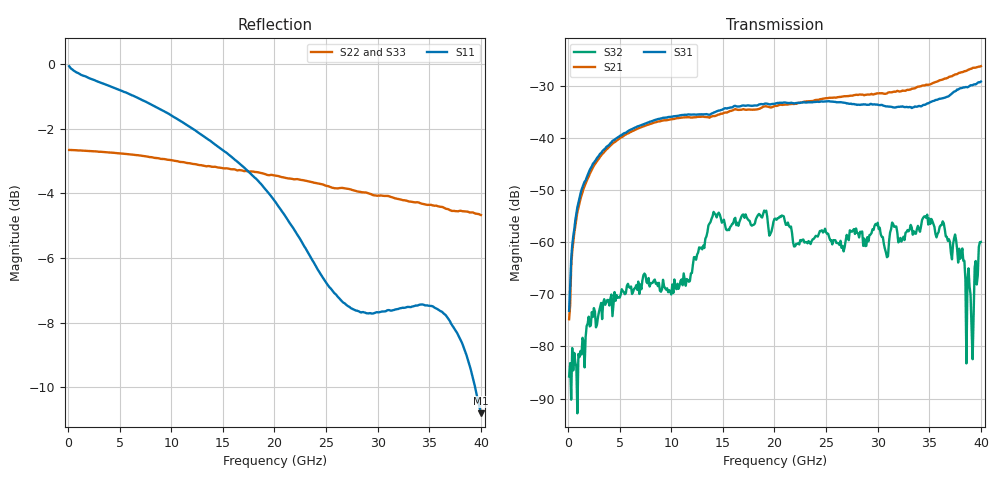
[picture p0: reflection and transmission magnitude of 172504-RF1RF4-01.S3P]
!  3-Port S-parameters saved by WinCal
! VAR MeasName=S-Parameters (CALIBRATED_DATA) read from VNA (N5245A)
! VAR MeasDate=2017-3-15 11:11:42
! VAR NAME=172504-RF1RF4-01
! VAR FILENAME=172504-RF1RF4-01.S3P
! VAR DATE=2017-3-15 11:11:42
! VAR PHYS_PORTS=1,2,3
# Hz S DB R 50
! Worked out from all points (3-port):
!   400 points, 100 MHz to 40 GHz, reference 50 ohm
!   strongest paths, dB at 100 MHz, 10.1 GHz, 20.1 GHz, 30.1 GHz, 40 GHz:
!     S31: -73.2, -35.9, -33.4, -33.7, -29.2
!     S21: -74.8, -36.4, -33.8, -31.4, -26.2
!     S32: -85.8, -68.1, -55.5, -57.5, -59.9
!   lowest |S11| = -10.8 dB at 40 GHz (marker M1), VSWR 1.81, Z = 29.5 - j10.8 ohm
!   |S11| at or under -10 dB: 39.44 GHz to end of sweep
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1e8  -0.06 -1.9  -91.03 159.2  -82.58 -148.7
     -74.78 102.3  -2.66 179.8  -90.02 167.2
     -73.17 86.1  -85.77 49.3  -2.64 179.8
8e8  -0.25 -12.4  -55.33 92.0  -54.34 90.6
     -55.53 93.0  -2.66 178.3  -80.38 96.8
     -54.54 90.9  -83.83 84.6  -2.65 178.3
3.4e9  -0.60 -48.0  -42.89 66.7  -42.33 64.1
       -42.91 67.0  -2.72 172.8  -73.01 69.8
       -42.35 64.1  -71.62 79.5  -2.70 173.0
1.19e10  -1.96 -140.4  -36.07 16.1  -35.50 13.6
         -36.06 16.0  -3.07 155.5  -66.18 118.0
         -35.49 13.6  -66.00 121.0  -3.03 155.8
2.01e10  -4.27 139.2  -33.81 -7.8  -33.31 -17.0
         -33.80 -7.2  -3.45 137.8  -55.60 37.1
         -33.36 -16.8  -55.48 38.3  -3.40 138.3
2.81e10  -7.64 16.0  -31.54 -39.9  -33.30 -53.9
         -31.72 -38.7  -3.94 118.2  -58.01 30.5
         -33.57 -52.2  -58.31 32.8  -3.92 118.5
3.63e10  -7.69 -93.8  -28.41 -71.4  -31.89 -69.2
         -28.76 -68.6  -4.42 94.6  -56.35 4.9
         -32.35 -66.1  -55.99 5.2  -4.56 94.4
3.82e10  -8.65 -117.9  -27.05 -83.1  -30.23 -77.2
         -27.34 -79.6  -4.55 88.9  -62.12 -22.0
         -30.36 -73.8  -61.19 -11.2  -4.71 88.3
3.86e10  -9.00 -123.3  -26.69 -86.3  -29.92 -80.5
         -27.07 -82.5  -4.56 87.5  -74.23 -127.0
         -30.20 -76.1  -83.25 -68.6  -4.75 86.9
4e10  -10.80 -144.5  -25.87 -97.2  -29.02 -87.8
      -26.19 -93.6  -4.67 82.6  -57.13 155.8
      -29.16 -82.1  -59.94 145.9  -4.83 82.9
